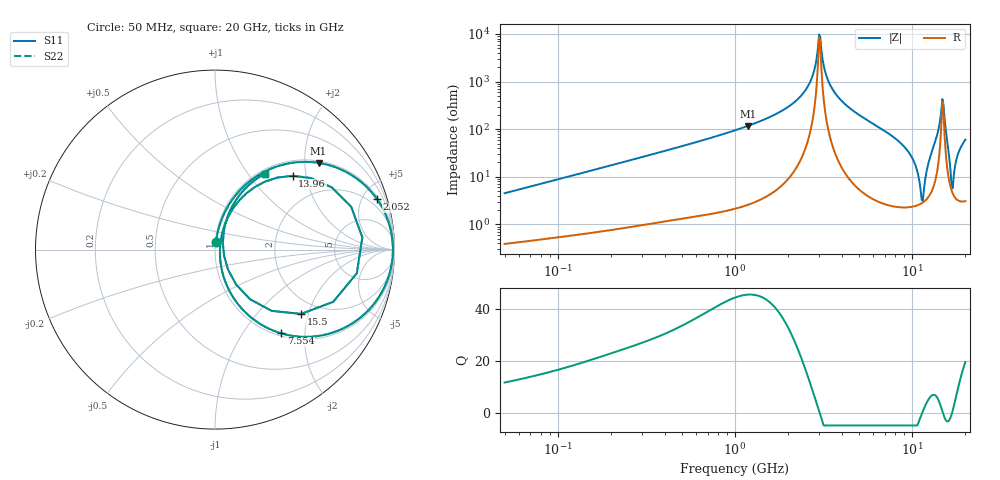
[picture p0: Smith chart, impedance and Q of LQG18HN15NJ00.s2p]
!Murata Part Number: LQG18HN15NJ00
!These Parameters are Measured in Series Mode Connection
!  o--[Z]--o
!Port1  Port2
!  o-------o
!Freq. Start=50[MHz] Stop=20[GHz], 401[Steps]
# Hz S RI R 50
!Freq.(Hz) S11(Real) S11(Imag) S21(Real) S21(Imag) S12(Real) S12(Imag) S22(Real) S22(Imag)
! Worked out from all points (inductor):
!   401 points, 50 MHz to 20 GHz, reference 50 ohm
!   read as one part in series: L = 14.2 nH near 51.52 MHz
!   highest Q = 45.6 at 1.179 GHz (marker M1), where L = 15.8 nH
!   self-resonance near 2.985 GHz
!   S11 on the Smith chart (normalised r, x): 50 MHz: 1.01, +0.09; 2.052 GHz: 1.20, +6.35; 7.554 GHz: 1.05, -1.52; 13.96 GHz: 1.31, +1.68; 15.5 GHz: 1.61, -1.80; 20 GHz: 1.06, +1.20
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5e7  0.00588 0.0446  0.9941 -0.0446  0.9941 -0.0446  0.00588 0.0446
1.364002e8  0.0201 0.1166  0.9799 -0.1166  0.9799 -0.1166  0.0201 0.1166
3.721004e8  0.1031 0.2876  0.8969 -0.2876  0.8969 -0.2876  0.1031 0.2876
1e9  0.4741 0.4882  0.5259 -0.4882  0.5259 -0.4882  0.4741 0.4882
1.179116e9  0.5768 0.4832  0.4232 -0.4832  0.4232 -0.4832  0.5768 0.4832
2.05233e9  0.9023 0.2813  0.0977 -0.2813  0.0977 -0.2813  0.9023 0.2813
2.728004e9  0.9851 0.0774  0.0149 -0.0774  0.0149 -0.0774  0.9851 0.0774
2.940159e9  0.9909 0.0172  0.00906 -0.0172  0.00906 -0.0172  0.9909 0.0172
3.029571e9  0.9912 -0.00724  0.00883 0.00724  0.00883 0.00724  0.9912 -0.00724
3.314454e9  0.9843 -0.0813  0.0157 0.0813  0.0157 0.0813  0.9843 -0.0813
3.850025e9  0.9465 -0.2036  0.0535 0.2036  0.0535 0.2036  0.9465 -0.2036
7.442007e9  0.3875 -0.4716  0.6125 0.4716  0.6125 0.4716  0.3875 -0.4716
7.554318e9  0.3697 -0.4668  0.6303 0.4668  0.6303 0.4668  0.3697 -0.4668
9.892087e9  0.0861 -0.2406  0.9139 0.2406  0.9139 0.2406  0.0861 -0.2406
1.131968e10  0.0274 -0.018  0.9726 0.018  0.9726 0.018  0.0274 -0.018
1.276073e10  0.1105 0.2436  0.8895 -0.2436  0.8895 -0.2436  0.1105 0.2436
1.396067e10  0.4329 0.4113  0.5671 -0.4113  0.5671 -0.4113  0.4329 0.4113
1.482269e10  0.8209 0.0684  0.1791 -0.0684  0.1791 -0.0684  0.8209 0.0684
1.550395e10  0.4797 -0.3584  0.5203 0.3584  0.5203 0.3584  0.4797 -0.3584
1.696185e10  0.044 0.0331  0.956 -0.0331  0.956 -0.0331  0.044 0.0331
1.828096e10  0.1156 0.2743  0.8844 -0.2743  0.8844 -0.2743  0.1156 0.2743
2e10  0.2764 0.4223  0.7236 -0.4223  0.7236 -0.4223  0.2764 0.4223
